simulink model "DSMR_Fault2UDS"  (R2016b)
settings: Solver=FixedStepDiscrete  StartTime=0.0  StopTime=10.0  FixedStep=0.02  RelTol=1e-3  EnableMultiTasking=on
undefined symbols (not defined in the file): bin2dec
libraries: simulink x312
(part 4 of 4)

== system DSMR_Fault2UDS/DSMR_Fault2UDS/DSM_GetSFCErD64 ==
  DFC : Inport  OutDataTypeStr=uint8
  DFC_IsoChkLv1_1 : simulink/Logic and Bit Operations/Bitwise Operator  logicop=AND  UseBitMask=on  BitMask=bin2dec('00011000')  BitMaskRealWorld=Stored Integer
  DFC_IsoChkLv1_1_compare : simulink/Logic and Bit Operations/Compare To Constant  relop===  const=24  OutDataTypeStr=boolean
  y : Outport
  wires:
  DFC_IsoChkLv1_1_compare/1 -> y/1
  DFC/1 -> DFC_IsoChkLv1_1/1
  DFC_IsoChkLv1_1/1 -> DFC_IsoChkLv1_1_compare/1

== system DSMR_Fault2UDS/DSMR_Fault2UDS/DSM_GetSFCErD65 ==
  DFC : Inport  OutDataTypeStr=uint8
  DFC_IsoChkLv1_1 : simulink/Logic and Bit Operations/Bitwise Operator  logicop=AND  UseBitMask=on  BitMask=bin2dec('00011000')  BitMaskRealWorld=Stored Integer
  DFC_IsoChkLv1_1_compare : simulink/Logic and Bit Operations/Compare To Constant  relop===  const=24  OutDataTypeStr=boolean
  y : Outport
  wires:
  DFC_IsoChkLv1_1_compare/1 -> y/1
  DFC/1 -> DFC_IsoChkLv1_1/1
  DFC_IsoChkLv1_1/1 -> DFC_IsoChkLv1_1_compare/1

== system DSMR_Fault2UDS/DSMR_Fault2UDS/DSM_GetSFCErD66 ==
  DFC : Inport  OutDataTypeStr=uint8
  DFC_IsoChkLv1_1 : simulink/Logic and Bit Operations/Bitwise Operator  logicop=AND  UseBitMask=on  BitMask=bin2dec('00011000')  BitMaskRealWorld=Stored Integer
  DFC_IsoChkLv1_1_compare : simulink/Logic and Bit Operations/Compare To Constant  relop===  const=24  OutDataTypeStr=boolean
  y : Outport
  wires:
  DFC_IsoChkLv1_1_compare/1 -> y/1
  DFC/1 -> DFC_IsoChkLv1_1/1
  DFC_IsoChkLv1_1/1 -> DFC_IsoChkLv1_1_compare/1

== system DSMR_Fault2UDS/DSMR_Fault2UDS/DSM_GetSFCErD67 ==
  DFC : Inport  OutDataTypeStr=uint8
  DFC_IsoChkLv1_1 : simulink/Logic and Bit Operations/Bitwise Operator  logicop=AND  UseBitMask=on  BitMask=bin2dec('00011000')  BitMaskRealWorld=Stored Integer
  DFC_IsoChkLv1_1_compare : simulink/Logic and Bit Operations/Compare To Constant  relop===  const=24  OutDataTypeStr=boolean
  y : Outport
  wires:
  DFC_IsoChkLv1_1_compare/1 -> y/1
  DFC/1 -> DFC_IsoChkLv1_1/1
  DFC_IsoChkLv1_1/1 -> DFC_IsoChkLv1_1_compare/1

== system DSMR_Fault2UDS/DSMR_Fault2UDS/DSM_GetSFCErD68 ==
  DFC : Inport  OutDataTypeStr=uint8
  DFC_IsoChkLv1_1 : simulink/Logic and Bit Operations/Bitwise Operator  logicop=AND  UseBitMask=on  BitMask=bin2dec('00011000')  BitMaskRealWorld=Stored Integer
  DFC_IsoChkLv1_1_compare : simulink/Logic and Bit Operations/Compare To Constant  relop===  const=24  OutDataTypeStr=boolean
  y : Outport
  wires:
  DFC_IsoChkLv1_1_compare/1 -> y/1
  DFC/1 -> DFC_IsoChkLv1_1/1
  DFC_IsoChkLv1_1/1 -> DFC_IsoChkLv1_1_compare/1

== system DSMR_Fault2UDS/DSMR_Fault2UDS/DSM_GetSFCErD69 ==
  DFC : Inport  OutDataTypeStr=uint8
  DFC_IsoChkLv1_1 : simulink/Logic and Bit Operations/Bitwise Operator  logicop=AND  UseBitMask=on  BitMask=bin2dec('00011000')  BitMaskRealWorld=Stored Integer
  DFC_IsoChkLv1_1_compare : simulink/Logic and Bit Operations/Compare To Constant  relop===  const=24  OutDataTypeStr=boolean
  y : Outport
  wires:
  DFC_IsoChkLv1_1_compare/1 -> y/1
  DFC/1 -> DFC_IsoChkLv1_1/1
  DFC_IsoChkLv1_1/1 -> DFC_IsoChkLv1_1_compare/1

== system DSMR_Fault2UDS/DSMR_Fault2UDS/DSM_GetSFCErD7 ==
  DFC : Inport  OutDataTypeStr=uint8
  DFC_IsoChkLv1_1 : simulink/Logic and Bit Operations/Bitwise Operator  logicop=AND  UseBitMask=on  BitMask=bin2dec('00011000')  BitMaskRealWorld=Stored Integer
  DFC_IsoChkLv1_1_compare : simulink/Logic and Bit Operations/Compare To Constant  relop===  const=24  OutDataTypeStr=boolean
  y : Outport
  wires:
  DFC_IsoChkLv1_1_compare/1 -> y/1
  DFC/1 -> DFC_IsoChkLv1_1/1
  DFC_IsoChkLv1_1/1 -> DFC_IsoChkLv1_1_compare/1

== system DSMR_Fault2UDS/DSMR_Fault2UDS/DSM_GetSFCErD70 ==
  DFC : Inport  OutDataTypeStr=uint8
  DFC_IsoChkLv1_1 : simulink/Logic and Bit Operations/Bitwise Operator  logicop=AND  UseBitMask=on  BitMask=bin2dec('00011000')  BitMaskRealWorld=Stored Integer
  DFC_IsoChkLv1_1_compare : simulink/Logic and Bit Operations/Compare To Constant  relop===  const=24  OutDataTypeStr=boolean
  y : Outport
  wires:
  DFC_IsoChkLv1_1_compare/1 -> y/1
  DFC/1 -> DFC_IsoChkLv1_1/1
  DFC_IsoChkLv1_1/1 -> DFC_IsoChkLv1_1_compare/1

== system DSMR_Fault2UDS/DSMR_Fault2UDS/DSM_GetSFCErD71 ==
  DFC : Inport  OutDataTypeStr=uint8
  DFC_IsoChkLv1_1 : simulink/Logic and Bit Operations/Bitwise Operator  logicop=AND  UseBitMask=on  BitMask=bin2dec('00011000')  BitMaskRealWorld=Stored Integer
  DFC_IsoChkLv1_1_compare : simulink/Logic and Bit Operations/Compare To Constant  relop===  const=24  OutDataTypeStr=boolean
  y : Outport
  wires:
  DFC_IsoChkLv1_1_compare/1 -> y/1
  DFC/1 -> DFC_IsoChkLv1_1/1
  DFC_IsoChkLv1_1/1 -> DFC_IsoChkLv1_1_compare/1

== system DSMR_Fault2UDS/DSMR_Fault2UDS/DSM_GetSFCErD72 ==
  DFC : Inport  OutDataTypeStr=uint8
  DFC_IsoChkLv1_1 : simulink/Logic and Bit Operations/Bitwise Operator  logicop=AND  UseBitMask=on  BitMask=bin2dec('00011000')  BitMaskRealWorld=Stored Integer
  DFC_IsoChkLv1_1_compare : simulink/Logic and Bit Operations/Compare To Constant  relop===  const=24  OutDataTypeStr=boolean
  y : Outport
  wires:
  DFC_IsoChkLv1_1_compare/1 -> y/1
  DFC/1 -> DFC_IsoChkLv1_1/1
  DFC_IsoChkLv1_1/1 -> DFC_IsoChkLv1_1_compare/1

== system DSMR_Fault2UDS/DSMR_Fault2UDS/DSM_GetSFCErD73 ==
  DFC : Inport  OutDataTypeStr=uint8
  DFC_IsoChkLv1_1 : simulink/Logic and Bit Operations/Bitwise Operator  logicop=AND  UseBitMask=on  BitMask=bin2dec('00011000')  BitMaskRealWorld=Stored Integer
  DFC_IsoChkLv1_1_compare : simulink/Logic and Bit Operations/Compare To Constant  relop===  const=24  OutDataTypeStr=boolean
  y : Outport
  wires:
  DFC_IsoChkLv1_1_compare/1 -> y/1
  DFC/1 -> DFC_IsoChkLv1_1/1
  DFC_IsoChkLv1_1/1 -> DFC_IsoChkLv1_1_compare/1

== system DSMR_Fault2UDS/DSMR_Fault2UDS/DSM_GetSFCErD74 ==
  DFC : Inport  OutDataTypeStr=uint8
  DFC_IsoChkLv1_1 : simulink/Logic and Bit Operations/Bitwise Operator  logicop=AND  UseBitMask=on  BitMask=bin2dec('00011000')  BitMaskRealWorld=Stored Integer
  DFC_IsoChkLv1_1_compare : simulink/Logic and Bit Operations/Compare To Constant  relop===  const=24  OutDataTypeStr=boolean
  y : Outport
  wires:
  DFC_IsoChkLv1_1_compare/1 -> y/1
  DFC/1 -> DFC_IsoChkLv1_1/1
  DFC_IsoChkLv1_1/1 -> DFC_IsoChkLv1_1_compare/1

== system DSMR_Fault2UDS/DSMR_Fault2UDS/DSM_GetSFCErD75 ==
  DFC : Inport  OutDataTypeStr=uint8
  DFC_IsoChkLv1_1 : simulink/Logic and Bit Operations/Bitwise Operator  logicop=AND  UseBitMask=on  BitMask=bin2dec('00011000')  BitMaskRealWorld=Stored Integer
  DFC_IsoChkLv1_1_compare : simulink/Logic and Bit Operations/Compare To Constant  relop===  const=24  OutDataTypeStr=boolean
  y : Outport
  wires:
  DFC_IsoChkLv1_1_compare/1 -> y/1
  DFC/1 -> DFC_IsoChkLv1_1/1
  DFC_IsoChkLv1_1/1 -> DFC_IsoChkLv1_1_compare/1

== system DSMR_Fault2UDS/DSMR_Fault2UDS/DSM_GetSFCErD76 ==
  DFC : Inport  OutDataTypeStr=uint8
  DFC_IsoChkLv1_1 : simulink/Logic and Bit Operations/Bitwise Operator  logicop=AND  UseBitMask=on  BitMask=bin2dec('00011000')  BitMaskRealWorld=Stored Integer
  DFC_IsoChkLv1_1_compare : simulink/Logic and Bit Operations/Compare To Constant  relop===  const=24  OutDataTypeStr=boolean
  y : Outport
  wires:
  DFC_IsoChkLv1_1_compare/1 -> y/1
  DFC/1 -> DFC_IsoChkLv1_1/1
  DFC_IsoChkLv1_1/1 -> DFC_IsoChkLv1_1_compare/1

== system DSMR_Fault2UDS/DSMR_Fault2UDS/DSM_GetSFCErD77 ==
  DFC : Inport  OutDataTypeStr=uint8
  DFC_IsoChkLv1_1 : simulink/Logic and Bit Operations/Bitwise Operator  logicop=AND  UseBitMask=on  BitMask=bin2dec('00011000')  BitMaskRealWorld=Stored Integer
  DFC_IsoChkLv1_1_compare : simulink/Logic and Bit Operations/Compare To Constant  relop===  const=24  OutDataTypeStr=boolean
  y : Outport
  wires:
  DFC_IsoChkLv1_1_compare/1 -> y/1
  DFC/1 -> DFC_IsoChkLv1_1/1
  DFC_IsoChkLv1_1/1 -> DFC_IsoChkLv1_1_compare/1

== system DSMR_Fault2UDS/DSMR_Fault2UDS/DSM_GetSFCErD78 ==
  DFC : Inport  OutDataTypeStr=uint8
  DFC_IsoChkLv1_1 : simulink/Logic and Bit Operations/Bitwise Operator  logicop=AND  UseBitMask=on  BitMask=bin2dec('00011000')  BitMaskRealWorld=Stored Integer
  DFC_IsoChkLv1_1_compare : simulink/Logic and Bit Operations/Compare To Constant  relop===  const=24  OutDataTypeStr=boolean
  y : Outport
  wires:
  DFC_IsoChkLv1_1_compare/1 -> y/1
  DFC/1 -> DFC_IsoChkLv1_1/1
  DFC_IsoChkLv1_1/1 -> DFC_IsoChkLv1_1_compare/1

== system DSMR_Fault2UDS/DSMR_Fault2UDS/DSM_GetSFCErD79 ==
  DFC : Inport  OutDataTypeStr=uint8
  DFC_IsoChkLv1_1 : simulink/Logic and Bit Operations/Bitwise Operator  logicop=AND  UseBitMask=on  BitMask=bin2dec('00011000')  BitMaskRealWorld=Stored Integer
  DFC_IsoChkLv1_1_compare : simulink/Logic and Bit Operations/Compare To Constant  relop===  const=24  OutDataTypeStr=boolean
  y : Outport
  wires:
  DFC_IsoChkLv1_1_compare/1 -> y/1
  DFC/1 -> DFC_IsoChkLv1_1/1
  DFC_IsoChkLv1_1/1 -> DFC_IsoChkLv1_1_compare/1

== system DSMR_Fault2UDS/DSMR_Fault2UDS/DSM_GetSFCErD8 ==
  DFC : Inport  OutDataTypeStr=uint8
  DFC_IsoChkLv1_1 : simulink/Logic and Bit Operations/Bitwise Operator  logicop=AND  UseBitMask=on  BitMask=bin2dec('00011000')  BitMaskRealWorld=Stored Integer
  DFC_IsoChkLv1_1_compare : simulink/Logic and Bit Operations/Compare To Constant  relop===  const=24  OutDataTypeStr=boolean
  y : Outport
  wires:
  DFC_IsoChkLv1_1_compare/1 -> y/1
  DFC/1 -> DFC_IsoChkLv1_1/1
  DFC_IsoChkLv1_1/1 -> DFC_IsoChkLv1_1_compare/1

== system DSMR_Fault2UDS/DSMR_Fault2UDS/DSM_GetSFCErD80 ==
  DFC : Inport  OutDataTypeStr=uint8
  DFC_IsoChkLv1_1 : simulink/Logic and Bit Operations/Bitwise Operator  logicop=AND  UseBitMask=on  BitMask=bin2dec('00011000')  BitMaskRealWorld=Stored Integer
  DFC_IsoChkLv1_1_compare : simulink/Logic and Bit Operations/Compare To Constant  relop===  const=24  OutDataTypeStr=boolean
  y : Outport
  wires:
  DFC_IsoChkLv1_1_compare/1 -> y/1
  DFC/1 -> DFC_IsoChkLv1_1/1
  DFC_IsoChkLv1_1/1 -> DFC_IsoChkLv1_1_compare/1

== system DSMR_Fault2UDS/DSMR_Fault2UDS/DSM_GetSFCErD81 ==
  DFC : Inport  OutDataTypeStr=uint8
  DFC_IsoChkLv1_1 : simulink/Logic and Bit Operations/Bitwise Operator  logicop=AND  UseBitMask=on  BitMask=bin2dec('00011000')  BitMaskRealWorld=Stored Integer
  DFC_IsoChkLv1_1_compare : simulink/Logic and Bit Operations/Compare To Constant  relop===  const=24  OutDataTypeStr=boolean
  y : Outport
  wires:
  DFC_IsoChkLv1_1_compare/1 -> y/1
  DFC/1 -> DFC_IsoChkLv1_1/1
  DFC_IsoChkLv1_1/1 -> DFC_IsoChkLv1_1_compare/1

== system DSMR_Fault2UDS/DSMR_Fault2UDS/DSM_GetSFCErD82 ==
  DFC : Inport  OutDataTypeStr=uint8
  DFC_IsoChkLv1_1 : simulink/Logic and Bit Operations/Bitwise Operator  logicop=AND  UseBitMask=on  BitMask=bin2dec('00011000')  BitMaskRealWorld=Stored Integer
  DFC_IsoChkLv1_1_compare : simulink/Logic and Bit Operations/Compare To Constant  relop===  const=24  OutDataTypeStr=boolean
  y : Outport
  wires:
  DFC_IsoChkLv1_1_compare/1 -> y/1
  DFC/1 -> DFC_IsoChkLv1_1/1
  DFC_IsoChkLv1_1/1 -> DFC_IsoChkLv1_1_compare/1

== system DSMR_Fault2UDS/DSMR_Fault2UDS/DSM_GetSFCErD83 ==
  DFC : Inport  OutDataTypeStr=uint8
  DFC_IsoChkLv1_1 : simulink/Logic and Bit Operations/Bitwise Operator  logicop=AND  UseBitMask=on  BitMask=bin2dec('00011000')  BitMaskRealWorld=Stored Integer
  DFC_IsoChkLv1_1_compare : simulink/Logic and Bit Operations/Compare To Constant  relop===  const=24  OutDataTypeStr=boolean
  y : Outport
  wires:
  DFC_IsoChkLv1_1_compare/1 -> y/1
  DFC/1 -> DFC_IsoChkLv1_1/1
  DFC_IsoChkLv1_1/1 -> DFC_IsoChkLv1_1_compare/1

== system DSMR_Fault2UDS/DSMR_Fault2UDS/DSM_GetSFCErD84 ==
  DFC : Inport  OutDataTypeStr=uint8
  DFC_IsoChkLv1_1 : simulink/Logic and Bit Operations/Bitwise Operator  logicop=AND  UseBitMask=on  BitMask=bin2dec('00011000')  BitMaskRealWorld=Stored Integer
  DFC_IsoChkLv1_1_compare : simulink/Logic and Bit Operations/Compare To Constant  relop===  const=24  OutDataTypeStr=boolean
  y : Outport
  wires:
  DFC_IsoChkLv1_1_compare/1 -> y/1
  DFC/1 -> DFC_IsoChkLv1_1/1
  DFC_IsoChkLv1_1/1 -> DFC_IsoChkLv1_1_compare/1

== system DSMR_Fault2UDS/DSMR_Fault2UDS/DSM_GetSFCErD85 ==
  DFC : Inport  OutDataTypeStr=uint8
  DFC_IsoChkLv1_1 : simulink/Logic and Bit Operations/Bitwise Operator  logicop=AND  UseBitMask=on  BitMask=bin2dec('00011000')  BitMaskRealWorld=Stored Integer
  DFC_IsoChkLv1_1_compare : simulink/Logic and Bit Operations/Compare To Constant  relop===  const=24  OutDataTypeStr=boolean
  y : Outport
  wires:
  DFC_IsoChkLv1_1_compare/1 -> y/1
  DFC/1 -> DFC_IsoChkLv1_1/1
  DFC_IsoChkLv1_1/1 -> DFC_IsoChkLv1_1_compare/1

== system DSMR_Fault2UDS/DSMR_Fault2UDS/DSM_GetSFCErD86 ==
  DFC : Inport  OutDataTypeStr=uint8
  DFC_IsoChkLv1_1 : simulink/Logic and Bit Operations/Bitwise Operator  logicop=AND  UseBitMask=on  BitMask=bin2dec('00011000')  BitMaskRealWorld=Stored Integer
  DFC_IsoChkLv1_1_compare : simulink/Logic and Bit Operations/Compare To Constant  relop===  const=24  OutDataTypeStr=boolean
  y : Outport
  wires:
  DFC_IsoChkLv1_1_compare/1 -> y/1
  DFC/1 -> DFC_IsoChkLv1_1/1
  DFC_IsoChkLv1_1/1 -> DFC_IsoChkLv1_1_compare/1

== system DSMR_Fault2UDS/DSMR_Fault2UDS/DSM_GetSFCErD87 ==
  DFC : Inport  OutDataTypeStr=uint8
  DFC_IsoChkLv1_1 : simulink/Logic and Bit Operations/Bitwise Operator  logicop=AND  UseBitMask=on  BitMask=bin2dec('00011000')  BitMaskRealWorld=Stored Integer
  DFC_IsoChkLv1_1_compare : simulink/Logic and Bit Operations/Compare To Constant  relop===  const=24  OutDataTypeStr=boolean
  y : Outport
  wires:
  DFC_IsoChkLv1_1_compare/1 -> y/1
  DFC/1 -> DFC_IsoChkLv1_1/1
  DFC_IsoChkLv1_1/1 -> DFC_IsoChkLv1_1_compare/1

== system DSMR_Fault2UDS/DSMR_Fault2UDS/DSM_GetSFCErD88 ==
  DFC : Inport  OutDataTypeStr=uint8
  DFC_IsoChkLv1_1 : simulink/Logic and Bit Operations/Bitwise Operator  logicop=AND  UseBitMask=on  BitMask=bin2dec('00011000')  BitMaskRealWorld=Stored Integer
  DFC_IsoChkLv1_1_compare : simulink/Logic and Bit Operations/Compare To Constant  relop===  const=24  OutDataTypeStr=boolean
  y : Outport
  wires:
  DFC_IsoChkLv1_1_compare/1 -> y/1
  DFC/1 -> DFC_IsoChkLv1_1/1
  DFC_IsoChkLv1_1/1 -> DFC_IsoChkLv1_1_compare/1

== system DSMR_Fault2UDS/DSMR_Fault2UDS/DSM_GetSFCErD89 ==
  DFC : Inport  OutDataTypeStr=uint8
  DFC_IsoChkLv1_1 : simulink/Logic and Bit Operations/Bitwise Operator  logicop=AND  UseBitMask=on  BitMask=bin2dec('00011000')  BitMaskRealWorld=Stored Integer
  DFC_IsoChkLv1_1_compare : simulink/Logic and Bit Operations/Compare To Constant  relop===  const=24  OutDataTypeStr=boolean
  y : Outport
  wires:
  DFC_IsoChkLv1_1_compare/1 -> y/1
  DFC/1 -> DFC_IsoChkLv1_1/1
  DFC_IsoChkLv1_1/1 -> DFC_IsoChkLv1_1_compare/1

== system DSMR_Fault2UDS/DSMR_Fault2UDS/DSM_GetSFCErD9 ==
  DFC : Inport  OutDataTypeStr=uint8
  DFC_IsoChkLv1_1 : simulink/Logic and Bit Operations/Bitwise Operator  logicop=AND  UseBitMask=on  BitMask=bin2dec('00011000')  BitMaskRealWorld=Stored Integer
  DFC_IsoChkLv1_1_compare : simulink/Logic and Bit Operations/Compare To Constant  relop===  const=24  OutDataTypeStr=boolean
  y : Outport
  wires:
  DFC_IsoChkLv1_1_compare/1 -> y/1
  DFC/1 -> DFC_IsoChkLv1_1/1
  DFC_IsoChkLv1_1/1 -> DFC_IsoChkLv1_1_compare/1

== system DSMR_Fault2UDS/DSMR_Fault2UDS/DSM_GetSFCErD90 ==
  DFC : Inport  OutDataTypeStr=uint8
  DFC_IsoChkLv1_1 : simulink/Logic and Bit Operations/Bitwise Operator  logicop=AND  UseBitMask=on  BitMask=bin2dec('00011000')  BitMaskRealWorld=Stored Integer
  DFC_IsoChkLv1_1_compare : simulink/Logic and Bit Operations/Compare To Constant  relop===  const=24  OutDataTypeStr=boolean
  y : Outport
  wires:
  DFC_IsoChkLv1_1_compare/1 -> y/1
  DFC/1 -> DFC_IsoChkLv1_1/1
  DFC_IsoChkLv1_1/1 -> DFC_IsoChkLv1_1_compare/1

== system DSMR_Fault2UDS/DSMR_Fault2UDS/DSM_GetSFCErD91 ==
  DFC : Inport  OutDataTypeStr=uint8
  DFC_IsoChkLv1_1 : simulink/Logic and Bit Operations/Bitwise Operator  logicop=AND  UseBitMask=on  BitMask=bin2dec('00011000')  BitMaskRealWorld=Stored Integer
  DFC_IsoChkLv1_1_compare : simulink/Logic and Bit Operations/Compare To Constant  relop===  const=24  OutDataTypeStr=boolean
  y : Outport
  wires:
  DFC_IsoChkLv1_1_compare/1 -> y/1
  DFC/1 -> DFC_IsoChkLv1_1/1
  DFC_IsoChkLv1_1/1 -> DFC_IsoChkLv1_1_compare/1

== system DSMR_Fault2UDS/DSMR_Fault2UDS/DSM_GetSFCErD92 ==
  DFC : Inport  OutDataTypeStr=uint8
  DFC_IsoChkLv1_1 : simulink/Logic and Bit Operations/Bitwise Operator  logicop=AND  UseBitMask=on  BitMask=bin2dec('00011000')  BitMaskRealWorld=Stored Integer
  DFC_IsoChkLv1_1_compare : simulink/Logic and Bit Operations/Compare To Constant  relop===  const=24  OutDataTypeStr=boolean
  y : Outport
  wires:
  DFC_IsoChkLv1_1_compare/1 -> y/1
  DFC/1 -> DFC_IsoChkLv1_1/1
  DFC_IsoChkLv1_1/1 -> DFC_IsoChkLv1_1_compare/1

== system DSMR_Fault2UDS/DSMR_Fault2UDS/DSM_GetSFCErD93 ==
  DFC : Inport  OutDataTypeStr=uint8
  DFC_IsoChkLv1_1 : simulink/Logic and Bit Operations/Bitwise Operator  logicop=AND  UseBitMask=on  BitMask=bin2dec('00011000')  BitMaskRealWorld=Stored Integer
  DFC_IsoChkLv1_1_compare : simulink/Logic and Bit Operations/Compare To Constant  relop===  const=24  OutDataTypeStr=boolean
  y : Outport
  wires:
  DFC_IsoChkLv1_1_compare/1 -> y/1
  DFC/1 -> DFC_IsoChkLv1_1/1
  DFC_IsoChkLv1_1/1 -> DFC_IsoChkLv1_1_compare/1

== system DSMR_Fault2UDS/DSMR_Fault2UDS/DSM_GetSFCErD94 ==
  DFC : Inport  OutDataTypeStr=uint8
  DFC_IsoChkLv1_1 : simulink/Logic and Bit Operations/Bitwise Operator  logicop=AND  UseBitMask=on  BitMask=bin2dec('00011000')  BitMaskRealWorld=Stored Integer
  DFC_IsoChkLv1_1_compare : simulink/Logic and Bit Operations/Compare To Constant  relop===  const=24  OutDataTypeStr=boolean
  y : Outport
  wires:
  DFC_IsoChkLv1_1_compare/1 -> y/1
  DFC/1 -> DFC_IsoChkLv1_1/1
  DFC_IsoChkLv1_1/1 -> DFC_IsoChkLv1_1_compare/1

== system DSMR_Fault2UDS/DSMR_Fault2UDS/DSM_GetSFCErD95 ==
  DFC : Inport  OutDataTypeStr=uint8
  DFC_IsoChkLv1_1 : simulink/Logic and Bit Operations/Bitwise Operator  logicop=AND  UseBitMask=on  BitMask=bin2dec('00011000')  BitMaskRealWorld=Stored Integer
  DFC_IsoChkLv1_1_compare : simulink/Logic and Bit Operations/Compare To Constant  relop===  const=24  OutDataTypeStr=boolean
  y : Outport
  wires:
  DFC_IsoChkLv1_1_compare/1 -> y/1
  DFC/1 -> DFC_IsoChkLv1_1/1
  DFC_IsoChkLv1_1/1 -> DFC_IsoChkLv1_1_compare/1

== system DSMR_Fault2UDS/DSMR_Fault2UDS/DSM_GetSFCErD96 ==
  DFC : Inport  OutDataTypeStr=uint8
  DFC_IsoChkLv1_1 : simulink/Logic and Bit Operations/Bitwise Operator  logicop=AND  UseBitMask=on  BitMask=bin2dec('00011000')  BitMaskRealWorld=Stored Integer
  DFC_IsoChkLv1_1_compare : simulink/Logic and Bit Operations/Compare To Constant  relop===  const=24  OutDataTypeStr=boolean
  y : Outport
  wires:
  DFC_IsoChkLv1_1_compare/1 -> y/1
  DFC/1 -> DFC_IsoChkLv1_1/1
  DFC_IsoChkLv1_1/1 -> DFC_IsoChkLv1_1_compare/1

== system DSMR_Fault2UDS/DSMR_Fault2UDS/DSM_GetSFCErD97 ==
  DFC : Inport  OutDataTypeStr=uint8
  DFC_IsoChkLv1_1 : simulink/Logic and Bit Operations/Bitwise Operator  logicop=AND  UseBitMask=on  BitMask=bin2dec('00011000')  BitMaskRealWorld=Stored Integer
  DFC_IsoChkLv1_1_compare : simulink/Logic and Bit Operations/Compare To Constant  relop===  const=24  OutDataTypeStr=boolean
  y : Outport
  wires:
  DFC_IsoChkLv1_1_compare/1 -> y/1
  DFC/1 -> DFC_IsoChkLv1_1/1
  DFC_IsoChkLv1_1/1 -> DFC_IsoChkLv1_1_compare/1

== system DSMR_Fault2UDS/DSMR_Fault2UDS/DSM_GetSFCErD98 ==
  DFC : Inport  OutDataTypeStr=uint8
  DFC_IsoChkLv1_1 : simulink/Logic and Bit Operations/Bitwise Operator  logicop=AND  UseBitMask=on  BitMask=bin2dec('00011000')  BitMaskRealWorld=Stored Integer
  DFC_IsoChkLv1_1_compare : simulink/Logic and Bit Operations/Compare To Constant  relop===  const=24  OutDataTypeStr=boolean
  y : Outport
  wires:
  DFC_IsoChkLv1_1_compare/1 -> y/1
  DFC/1 -> DFC_IsoChkLv1_1/1
  DFC_IsoChkLv1_1/1 -> DFC_IsoChkLv1_1_compare/1

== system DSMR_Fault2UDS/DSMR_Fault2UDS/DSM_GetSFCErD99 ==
  DFC : Inport  OutDataTypeStr=uint8
  DFC_IsoChkLv1_1 : simulink/Logic and Bit Operations/Bitwise Operator  logicop=AND  UseBitMask=on  BitMask=bin2dec('00011000')  BitMaskRealWorld=Stored Integer
  DFC_IsoChkLv1_1_compare : simulink/Logic and Bit Operations/Compare To Constant  relop===  const=24  OutDataTypeStr=boolean
  y : Outport
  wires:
  DFC_IsoChkLv1_1_compare/1 -> y/1
  DFC/1 -> DFC_IsoChkLv1_1/1
  DFC_IsoChkLv1_1/1 -> DFC_IsoChkLv1_1_compare/1
